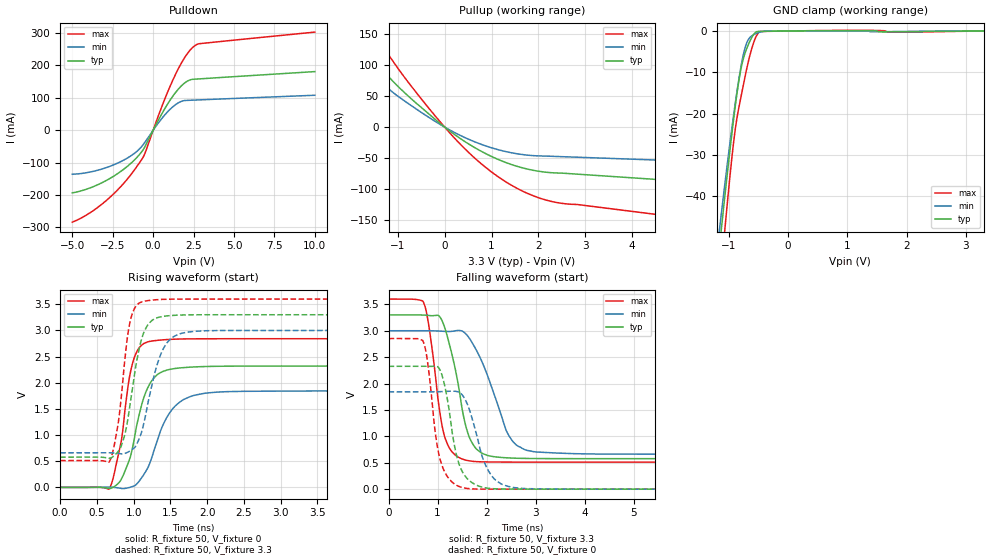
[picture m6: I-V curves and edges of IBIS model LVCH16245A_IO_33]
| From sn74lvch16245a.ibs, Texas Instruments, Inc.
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[Model]   LVCH16245A_IO_33
Model_type  3-state
Enable   Active-Low
Vref =   0
Rref =   500
Cref =   50p
Vmeas =   1.5
| variable   typ   min   max
C_comp   4.45pF   3.96pF   5.50pF
| C_pullup   6.29pF   3.94pF   9.02pF
| C_pulldown   6.69pF   4.45pF   8.68pF
| C_tri-state   4.45pF   3.96pF   5.50pF
[Temperature Range]   40   100   -40
| Ambient temperature   25   85   -40
[Voltage range]   3.3   3   3.6
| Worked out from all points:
|   slope of the pulldown table from 0 to 0.495 V, typ, clamps not added: 10.5 ohm
|   slope of the pullup table from 0 to 0.495 V, typ, clamps not added: 18.8 ohm
|   GND clamp passes 1 mA (typ) near -0.59 V on its own axis
|   rising waveform, R_fixture 50, V_fixture 0: 20-80 % time 251ps typ, 325ps min, 184ps max; typ from 0 V to 2.32 V
|   falling waveform, R_fixture 50, V_fixture 3.3: 20-80 % time 360ps typ, 546ps min, 268ps max; typ from 3.3 V to 0.577 V
|   rising waveform, R_fixture 50, V_fixture 3.3: 20-80 % time 195ps typ, 244ps min, 149ps max; typ from 0.577 V to 3.3 V
|   falling waveform, R_fixture 50, V_fixture 0: 20-80 % time 275ps typ, 365ps min, 235ps max; typ from 2.33 V to 0 V
[GND Clamp]
| LVCH16245A_IO_33
|   Voltage   I(typ)   I(min)   I(max)
-5V       -658mA     -597.1mA   -758.8mA
-1.165V   -53.49mA   -49.12mA   -63.76mA
-1.13V    -48.68mA   -44.82mA   -58.16mA
-1.095V   -43.94mA   -40.58mA   -52.63mA
-1.065V   -39.92mA   -37mA      -47.96mA
-900mV    -19.31mA   -18.52mA   -24.88mA
-790mV    -8.892mA   -8.331mA   -15.66mA
-730mV    -5.567mA   -4.352mA   -11.4mA
-675mV    -3.469mA   -2.205mA   -7.757mA
-580mV    -839.4uA   -901.1uA   -2.808mA
-485mV    -96.87uA   -311.8uA   -253.4uA
3.3V      17.26pA    96.68nA    -142.7nA
[Pulldown]
| LVCH16245A_IO_33
|   Voltage   I(typ)   I(min)   I(max)
-5V       -193.4mA   -135.8mA   -283.8mA
-3.865V   -177.3mA   -128.6mA   -253.5mA
-2.715V   -149.9mA   -112mA     -208.9mA
-1.535V   -108.9mA   -83.98mA   -147.1mA
-730mV    -67.77mA   -51.47mA   -92.05mA
-485mV    -48.43mA   -35.35mA   -68.52mA
485mV     46.17mA    33.18mA    66.28mA
1.245V    107.2mA    73.64mA    157.8mA
1.945V    145.9mA    91.78mA    224mA
2.535V    157.6mA    93.17mA    259.6mA
2.87V     158.7mA    93.86mA    267.5mA
10V       181.2mA    108.1mA    303.1mA
[Pullup]
| LVCH16245A_IO_33
|   Voltage   I(typ)   I(min)   I(max)
-5V       411.3mA    305.7mA    585.7mA
-2.62V    205.7mA    159.3mA    291mA
-2.225V   170.4mA    131.7mA    241.6mA
-2.015V   151.8mA    117.1mA    215.6mA
-1.6V     115.4mA    88.61mA    163.8mA
-735mV    47.21mA    35.83mA    68.13mA
-100mV    6.049mA    4.476mA    8.826mA
425mV     -23.01mA   -16.64mA   -34.51mA
1.32V     -57.53mA   -39.73mA   -88.97mA
2.135V    -72.53mA   -46.66mA   -117.1mA
6.505V    -94.5mA    -58.51mA   -159.8mA
10V       -112.3mA   -68.03mA   -193.4mA
[Ramp]
| LVCH16245A_IO_33
| variable   typ   min   max
dV/dt_r   1.41/2.61E-10   1.12/3.35E-10   1.73/1.90E-10
dV/dt_f   1.63/3.61E-10   1.41/5.52E-10   1.85/2.76E-10
R_load = 50
[Rising Waveform]
| LVCH16245A_IO_33
R_fixture =   50
C_fixture =   0
L_fixture =   0
V_fixture =   0
V_fixture_min = 0
V_fixture_max = 0
|   Time   V(typ)   V(min)   V(max)
0s        -15.15uV   -29.34uV   -5.769uV
665ps     -19.76mV   4.843mV    -32.26mV
845ps     192.9mV    -22.89mV   1.016V
935ps     501.9mV    -4.577mV   2.041V
1.02ns    1.018V     37.87mV    2.523V
1.225ns   1.993V     485mV      2.792V
1.54ns    2.268V     1.518V     2.832V
1.975ns   2.31V      1.8V       2.841V
3.215ns   2.319V     1.842V     2.842V
50ns      2.319V     1.844V     2.842V
[Falling Waveform]
| LVCH16245A_IO_33
R_fixture =   50
C_fixture =   0
L_fixture =   0
V_fixture =   3.3
V_fixture_min = 3
V_fixture_max = 3.6
|   Time   V(typ)   V(min)   V(max)
0s        3.3V       3V         3.6V
715ps     3.297V     3V         3.532V
835ps     3.288V     2.999V     3.014V
1.06ns    3.244V     2.993V     1.373V
1.29ns    2.565V     2.989V     712.9mV
1.575ns   1.197V     2.941V     550.1mV
1.795ns   757.8mV    2.624V     521.5mV
2.53ns    588.4mV    909.3mV    512.7mV
3.45ns    578.2mV    683.3mV    512.1mV
50ns      577.4mV    661.5mV    512.1mV
[Rising Waveform]
| LVCH16245A_IO_33
R_fixture =   50
C_fixture =   0
L_fixture =   0
V_fixture =   3.3
V_fixture_min = 3
V_fixture_max = 3.6
|   Time   V(typ)   V(min)   V(max)
0s        577.4mV    661.4mV    512.1mV
665ps     558.7mV    661.9mV    482.7mV
765ps     647.4mV    652.7mV    1.026V
840ps     828.8mV    639.6mV    1.85V
975ps     1.809V     719.5mV    3.295V
1.135ns   2.949V     1.206V     3.555V
1.37ns    3.26V      2.549V     3.592V
1.62ns    3.294V     2.932V     3.599V
2.19ns    3.3V       2.999V     3.6V
50ns      3.3V       3V         3.6V
[Falling Waveform]
| LVCH16245A_IO_33
R_fixture =   50
C_fixture =   0
L_fixture =   0
V_fixture =   0
V_fixture_min = 0
V_fixture_max = 0
|   Time   V(typ)   V(min)   V(max)
0s        2.326V     1.843V     2.853V
700ps     2.327V     1.843V     2.81V
795ps     2.327V     1.843V     2.413V
1.02ns    2.303V     1.846V     686mV
1.16ns    1.894V     1.851V     300.1mV
1.41ns    558.6mV    1.845V     62.35mV
1.705ns   121.5mV    1.335V     5.259mV
2.115ns   9.972mV    237.1mV    1.022mV
2.815ns   857.7uV    9.827mV    204.4uV
50ns      7.631uV    34.65uV    5.235uV
